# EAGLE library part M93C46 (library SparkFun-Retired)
Datasheet SparkFun Products () () 1kbit SPI EEPROM IC-09397 -- Dead prototype
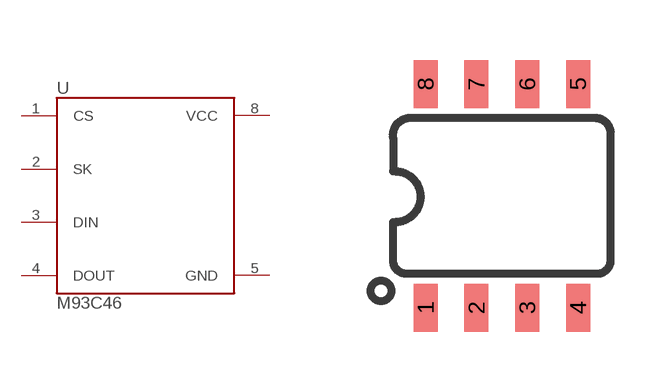
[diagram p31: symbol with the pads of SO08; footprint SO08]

Designator prefix -

## M93C46  [SO08]
1  CS
2  SK
3  DIN
4  DOUT
5  GND
8  VCC

## Footprint SO08 (pad centres in mm)
SOIC, 0.15 inch width
smd 0.6 x 1.2: 1 -1.905,-2.8; 2 -0.635,-2.8; 3 0.635,-2.8; 4 1.905,-2.8; 5 1.905,2.8; 6 0.635,2.8; 7 -0.635,2.8; 8 -1.905,2.8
